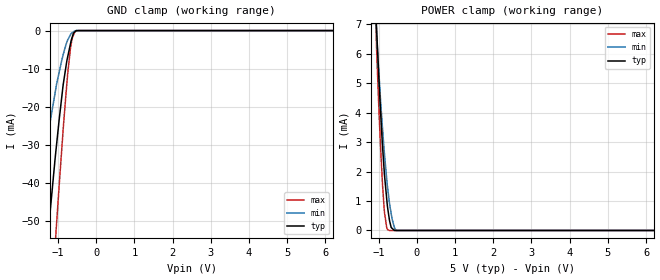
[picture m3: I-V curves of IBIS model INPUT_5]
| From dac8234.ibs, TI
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|   input_5 Model
[Model]   INPUT_5
Model_type   Input
Vinl = 0.6
Vinh = 2.5
|   typ   min   max
|   (nom PVT)   (Fast PVT)   (slow PVT)
|Average
C_comp   2.504e-12   1.971e-12   2.935e-12
[Voltage Range]   5   4.5   5.5
|Ambient Temperature   25   105   -40
|Junction Temperature
[Temperature Range]   42   122   -40
[Power Clamp Reference]   5   4.5   5.5
[GND Clamp Reference]   0   0   0
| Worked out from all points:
|   GND clamp passes 1 mA (typ) near -0.60 V on its own axis
|   POWER clamp passes 1 mA (typ) near -0.78 V on its own axis
[GND Clamp]
|   Voltage   I(typ)   I(min)   I(max)
-5V       -564.1mA   -401mA     -700.8mA
-1.735V   -111.9mA   -63.43mA   -163mA
-1.59V    -93.42mA   -51.59mA   -139.1mA
-1.391V   -69.04mA   -36.53mA   -106.6mA
-1.244V   -51.92mA   -26.45mA   -82.87mA
-1.051V   -31.39mA   -15mA      -52.93mA
-865mV    -14.41mA   -6.421mA   -26.24mA
-743mV    -6.808mA   -2.428mA   -11.21mA
-655mV    -2.692mA   -812.8uA   -3.565mA
-622mV    -1.595mA   -518.6uA   -1.914mA
-556mV    -355.2uA   -83.02uA   -237.1uA
10V       0A         0A         0A
[POWER Clamp]
|   Voltage   I(typ)   I(min)   I(max)
-5V       170.1mA    141.7mA    212mA
-1.07V    7.376mA    7.216mA    6.975mA
-1.065V   7.224mA    7.085mA    6.752mA
-1.046V   6.676mA    6.572mA    5.961mA
-952mV    4.142mA    4.51mA     2.967mA
-897mV    2.885mA    3.473mA    1.578mA
-853mV    2.039mA    2.724mA    731uA
-787mV    1.079mA    1.75mA     108.5uA
-716mV    363.6uA    943.9uA    0A
-644mV    69.21uA    382.5uA    0A
-535mV    0A         0A         0A
10V       0A         0A         0A
